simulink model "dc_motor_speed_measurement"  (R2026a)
settings: Solver=FixedStepAuto  StopTime=inf  EnableMultiTasking=on
libraries: arduinosensorlib x1, arduinolib x1

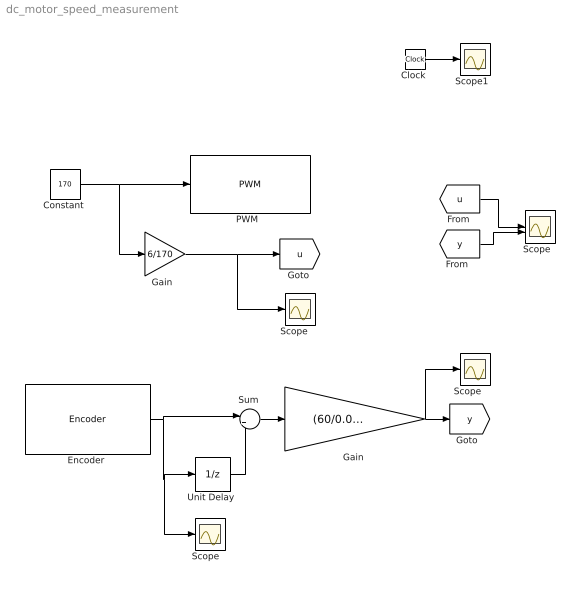
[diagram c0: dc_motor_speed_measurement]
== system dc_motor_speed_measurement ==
  "Clock " : Clock
  "Constant " : Constant  Value=170
  "Encoder " : arduinosensorlib/Encoder  InputA=2  InputB=3  Mode=No reset  SampleTime=0.01
  "Gain " : Gain  Gain=(60/0.01)*(1/(12*298))
  "Gain  " : Gain  Gain=6/170
  "PWM  " : arduinolib/PWM  pinNumber=5  frequencyType=Default  desiredFrequency=490.2  achievableFrequency=490.2
  "Scope  " : Scope  NumInputPorts=2
  "Scope   " : Scope
  "Scope    " : Scope
  "Scope     " : Scope
  "Scope1  " : Scope
  "Sum " : Sum  Inputs=|+-
  "Unit Delay " : UnitDelay  SampleTime=-1
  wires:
  "Encoder "/1 -> "Sum "/1, "Scope   "/1, "Unit Delay "/1
  "Sum "/1 -> "Gain "/1
  "Unit Delay "/1 -> "Sum "/2
  "Constant "/1 -> "PWM  "/1, "Gain  "/1
  "Gain "/1 -> "Scope     "/1, [y]
  "Gain  "/1 -> "Scope    "/1, [u]
  [u] -> "Scope  "/1
  [y] -> "Scope  "/2
  "Clock "/1 -> "Scope1  "/1
